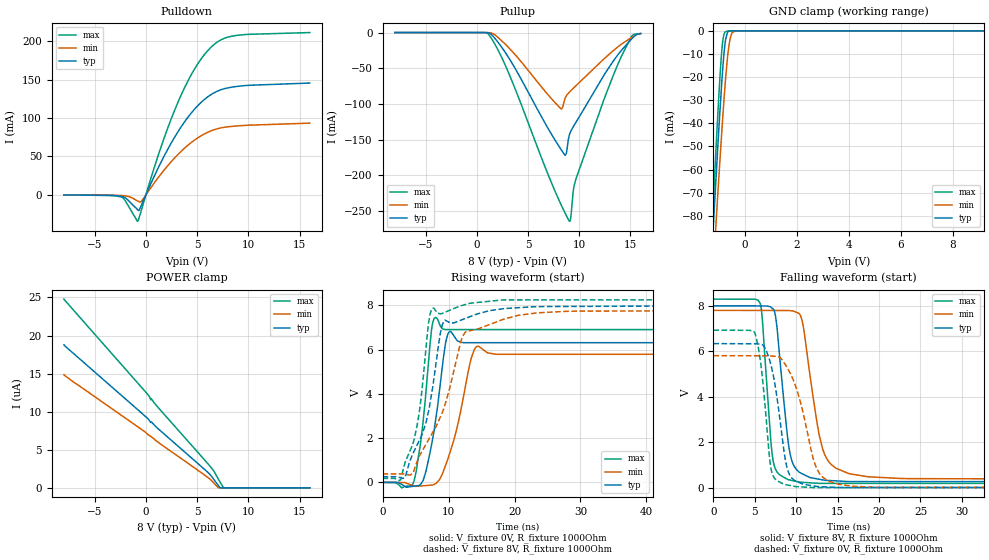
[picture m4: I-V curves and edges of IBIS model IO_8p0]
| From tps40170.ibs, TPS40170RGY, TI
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|   IO_8p0 Model
[Model]   IO_8p0
Model_type   I/O
Polarity   Non-Inverting
Enable   Active-High
Vinl = 0.8
Vinh = 2
Vmeas = 4
Vref = 0
Cref = 2pF
Rref = 100000
|   typ   min   max
C_comp   2.206E-12   1.878E-12   2.241E-12
|  Where Nom  PVT is Nominal Process, 8.0V,  27C
|   Fast PVT is Strong Process,  8.3V, -40C
|   Slow PVT is Weak Process,   7.8V, 125C
[Voltage Range]   8   7.8   8.3
|Junction Temperature
[Temperature Range]   27   125   -40
[Pullup Reference]   8   7.8   8.3
[Pulldown Reference]   0   0   0
[Power Clamp Reference]   8   7.8   8.3
[GND Clamp Reference]   0   0   0
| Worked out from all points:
|   slope of the pulldown table from 0 to 1.2 V, typ, clamps not added: 34.3 ohm
|   slope of the pullup table from 0 to 1.2 V, typ, clamps not added: 1.73 kohm
|   GND clamp passes 1 mA (typ) near -0.66 V on its own axis
|   falling waveform, V_fixture 8V, R_fixture 1000Ohm: 20-80 % time 1.28ns typ, 1.92ns min, 952ps max; typ from 7.99 V to 0.254 V
|   rising waveform, V_fixture 0V, R_fixture 1000Ohm: 20-80 % time 1.85ns typ, 2.74ns min, 1.43ns max; typ from 0 V to 6.33 V
|   rising waveform, V_fixture 8V, R_fixture 1000Ohm: 20-80 % time 3.19ns typ, 4.96ns min, 2.11ns max; typ from 0.254 V to 7.99 V
|   falling waveform, V_fixture 0V, R_fixture 1000Ohm: 20-80 % time 1.51ns typ, 2.41ns min, 1.07ns max; typ from 6.33 V to 0 V
[Pulldown]
|   Voltage   I(typ)   I(min)   I(max)
-8V       -115.2uA   -80.17uA   -134.7uA
-2.408V   -1.863mA   -919.9uA   -2.756mA
-824mV    -19.27mA   -7.926mA   -34.47mA
-656mV    -19.78mA   -9.218mA   -29.39mA
-440mV    -13.55mA   -8.566mA   -19.82mA
1.36V     39.34mA    25.17mA    57.76mA
3.04V     80.2mA     51.3mA     117.7mA
4.72V     111.1mA    70.97mA    163.1mA
6.064V    127.8mA    81.53mA    188mA
7.288V    136.6mA    87.02mA    201.5mA
8.416V    140.2mA    89.1mA     206.5mA
16V       145.5mA    93.29mA    211.2mA
[GND Clamp]
|   Voltage   I(typ)   I(min)   I(max)
-8V       -1.552A    -1.463A    -1.686A
-1.256V   -95.66mA   -112.9mA   -85.93mA
-1.184V   -80.98mA   -99.34mA   -69.75mA
-1.136V   -71.31mA   -90.37mA   -59.11mA
-1.04V    -52.34mA   -72.66mA   -38.44mA
-872mV    -21.63mA   -42.97mA   -7.958mA
-824mV    -14.19mA   -35mA      -3.256mA
-752mV    -5.637mA   -23.84mA   -599.5uA
-656mV    -676.8uA   -11.48mA   -84.73uA
-536mV    -14.45uA   -2.528mA   -4.266uA
-320mV    0A         -13.42uA   0A
16V       0A         0A         0A
[Pullup]
|   Voltage   I(typ)   I(min)   I(max)
-8V       3.55nA     14.16nA    776.7pA
1.168V    -453.5uA   -105.2uA   -2.704mA
3.112V    -35.13mA   -21.07mA   -56.68mA
8.176V    -162.8mA   -106.3mA   -239.6mA
8.608V    -171.9mA   -92.8mA    -252.7mA
9.088V    -141.6mA   -82.93mA   -264.7mA
9.208V    -137.6mA   -81.2mA    -256.1mA
9.424V    -132mA     -78.18mA   -222.3mA
9.664V    -126.3mA   -74.86mA   -206.4mA
12.54V    -56.96mA   -35.34mA   -89.15mA
15.14V    -8.586mA   -6.708mA   -4.663mA
16V       -1.455mA   -1.377mA   -1.352mA
[POWER Clamp]
|   Voltage   I(typ)   I(min)   I(max)
-8V       18.77uA    14.87uA    24.78uA
88mV      9.212uA    7.139uA    12.4uA
352mV     8.823uA    6.86uA     11.94uA
472mV     8.594uA    6.753uA    11.55uA
496mV     8.672uA    6.73uA     11.73uA
1V        7.996uA    6.18uA     10.85uA
6.256V    1.749uA    1.141uA    2.846uA
6.64V     1.084uA    616.8nA    2.176uA
7.072V    309.5nA    25.83nA    1.153uA
7.24V     35.12nA    0A         758.5nA
7.576V    0A         0A         25.59nA
16V       0A         0A         0A
[Ramp]
R_load = 1000
|   typ   min   max
dV/dt_r   3.80061/1.85643e-09   3.48312/2.72164e-09   4.15453/1.42992e-09
dV/dt_f   4.64168/1.27735e-09   4.44581/1.90093e-09   4.86393/9.51298e-10
[Falling Waveform]
V_fixture = 8V
V_fixture_min = 7.8V
V_fixture_max = 8.3V
R_fixture = 1000Ohm
C_fixture = 0F
|   Time   V(typ)   V(min)   V(max)
0s        7.99V      7.792V     8.287V
5.665ns   7.989V     7.791V     8.082V
6.979ns   7.923V     7.79V      1.904V
7.292ns   7.822V     7.79V      1.057V
9.141ns   1.74V      7.786V     352.5mV
10.4ns    675.7mV    7.633V     254.6mV
12.77ns   377.4mV    2.335V     197.5mV
14.82ns   306.2mV    856.2mV    197.5mV
23.47ns   275.2mV    405.8mV    197.3mV
833.4ns   254.3mV    382.8mV    180.7mV
[Rising Waveform]
V_fixture = 0V
V_fixture_min = 0V
V_fixture_max = 0V
R_fixture = 1000Ohm
C_fixture = 0F
|   Time   V(typ)   V(min)   V(max)
0s        -621.2nV   3.219uV    -395.5nV
4.795ns   -172.9mV   -169.4mV   79.56mV
6.17ns    101.1mV    -154.8mV   2.82V
7.399ns   1.653V     -124.8mV   6.831V
8.015ns   2.754V     -61.99mV   7.458V
9.916ns   6.716V     1.07V      6.909V
11.3ns    6.415V     2.477V     6.909V
13.36ns   6.317V     5.517V     6.909V
14.39ns   6.317V     6.158V     6.91V
833.4ns   6.334V     5.805V     6.924V
[Rising Waveform]
V_fixture = 8V
V_fixture_min = 7.8V
V_fixture_max = 8.3V
R_fixture = 1000Ohm
C_fixture = 0F
|   Time   V(typ)   V(min)   V(max)
0s        254.3mV    382.8mV    180.7mV
2.726ns   210.9mV    382.2mV    108.8mV
4.696ns   1.355V     478.1mV    1.836V
5.6ns     1.914V     1.203V     3.239V
6.922ns   3.153V     1.899V     7.088V
7.446ns   4.028V     2.175V     7.83V
9.332ns   7.31V      3.391V     7.678V
12.53ns   7.411V     6.788V     8.04V
18.28ns   7.853V     7.372V     8.253V
833.4ns   7.99V      7.792V     8.287V
[Falling Waveform]
|Gnd
V_fixture = 0V
V_fixture_min = 0V
V_fixture_max = 0V
R_fixture = 1000Ohm
C_fixture = 0F
|   Time   V(typ)   V(min)   V(max)
0s        6.334V     5.805V     6.924V
4.96ns    6.326V     5.799V     6.834V
6.119ns   6.218V     5.798V     4.092V
6.807ns   5.592V     5.794V     1.224V
7.259ns   4.892V     5.783V     492.5mV
9.04ns    708.1mV    5.19V      117.9mV
12.02ns   87.64mV    1.325V     13.35mV
13.83ns   36.5mV     306.5mV    13.32mV
20.02ns   14.67mV    20.21mV    13.22mV
833.4ns   -545.7nV   3.249uV    -396nV
